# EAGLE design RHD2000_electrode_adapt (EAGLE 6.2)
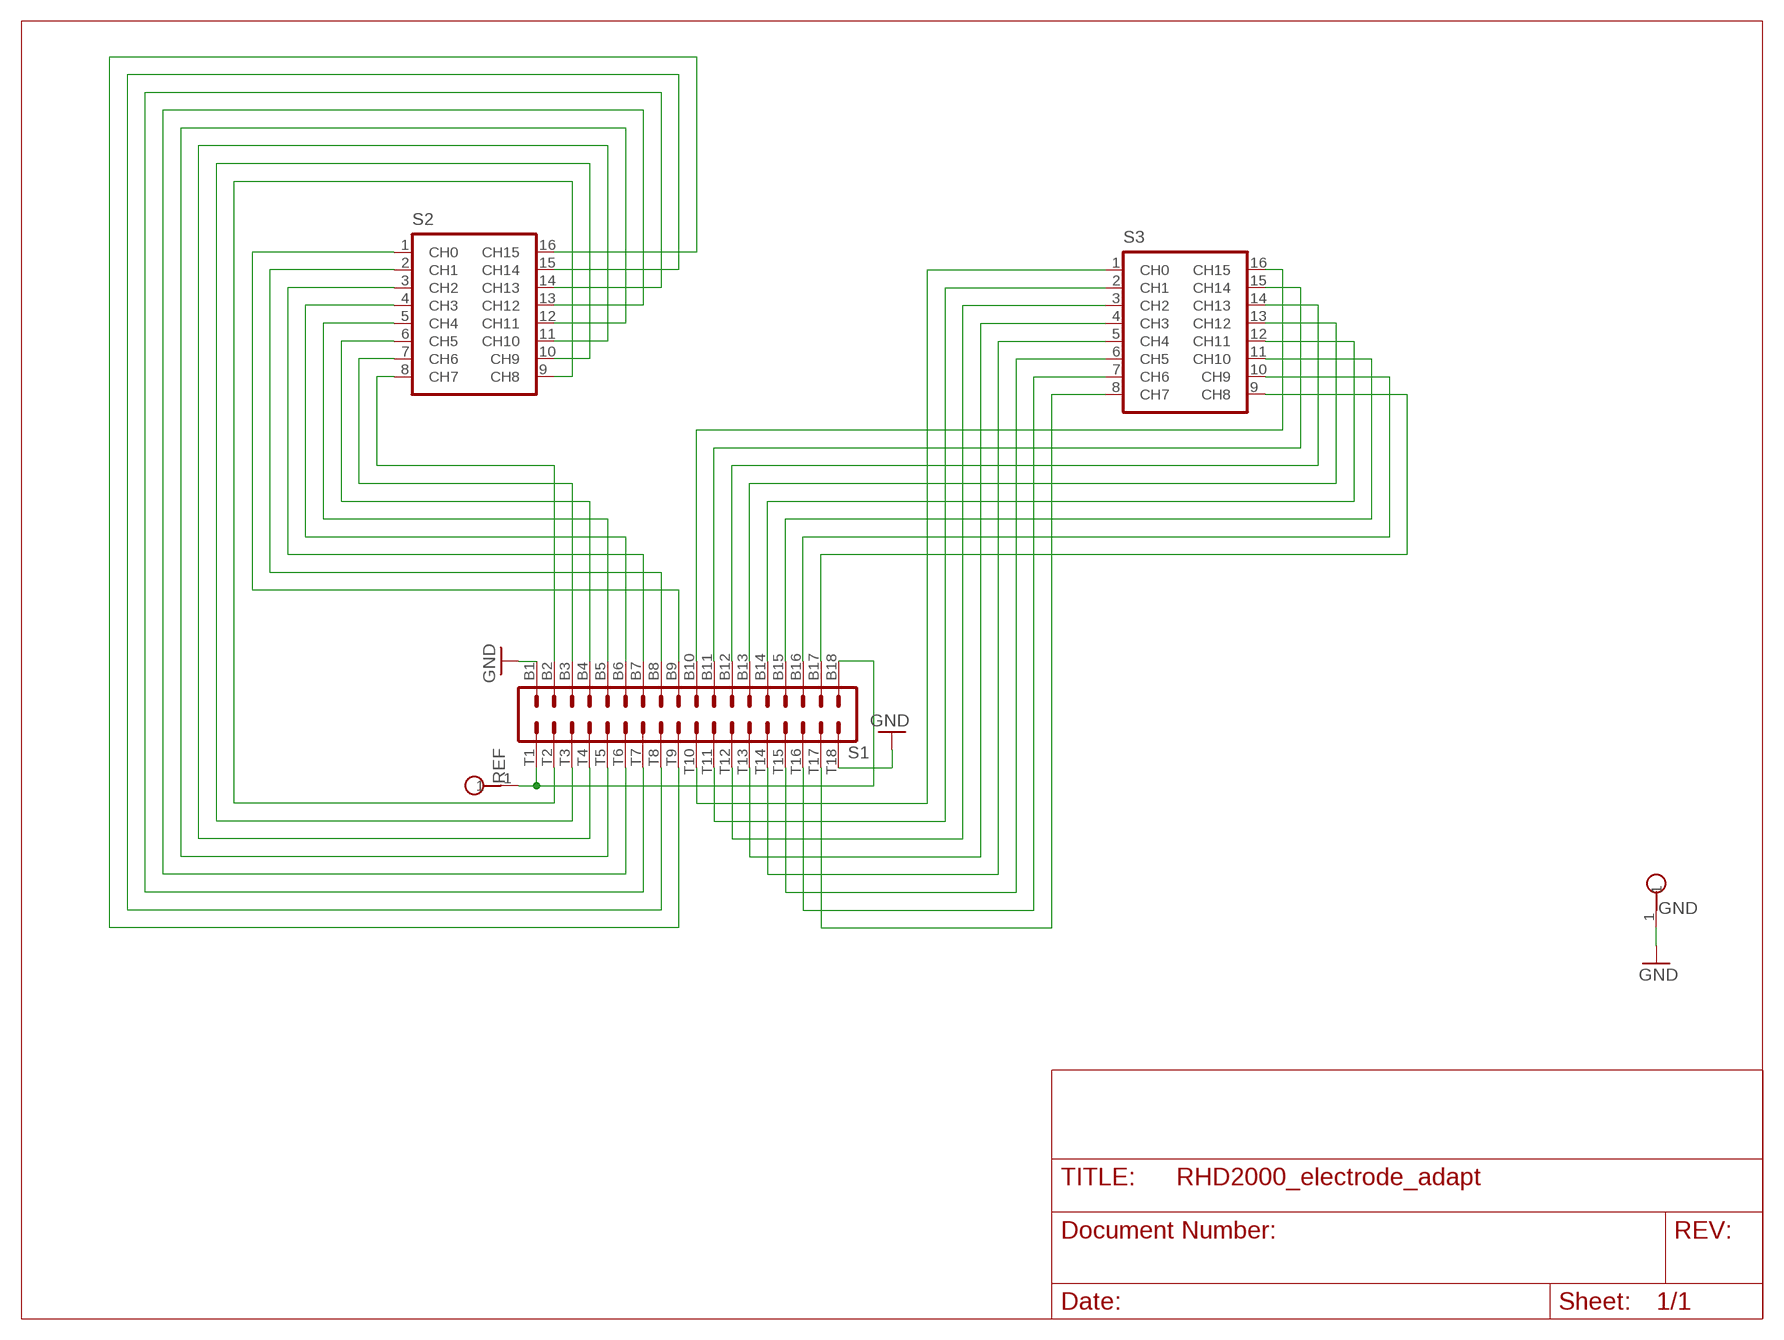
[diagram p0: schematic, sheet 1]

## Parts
GND  TESTPOINT_SMALL  [TESTPOINT_SMALL]
REF  TESTPOINT_SMALL  [TESTPOINT_SMALL]
S1  OMNETICS_A79024  [OMNETICS_A79024]
S2  DIP16_SOCKET  [DIL16_SOCKET]
S3  DIP16_SOCKET  [DIL16_SOCKET]

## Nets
GND: GND.1 S1.B1 S1.T18
N$1: REF.1 S1.B18 S1.T1
N$2: S1.B2 S2.8(CH7)
N$3: S1.B3 S2.7(CH6)
N$4: S1.B4 S2.6(CH5)
N$5: S1.B5 S2.5(CH4)
N$6: S1.B6 S2.4(CH3)
N$7: S1.B7 S2.3(CH2)
N$8: S1.B8 S2.2(CH1)
N$9: S1.B9 S2.1(CH0)
N$10: S1.T2 S2.9(CH8)
N$11: S1.T3 S2.10(CH9)
N$12: S1.T4 S2.11(CH10)
N$13: S1.T5 S2.12(CH11)
N$14: S1.T6 S2.13(CH12)
N$15: S1.T7 S2.14(CH13)
N$16: S1.T8 S2.15(CH14)
N$17: S1.T9 S2.16(CH15)
N$18: S1.T10 S3.1(CH0)
N$19: S1.T11 S3.2(CH1)
N$20: S1.T12 S3.3(CH2)
N$21: S1.T13 S3.4(CH3)
N$22: S1.T14 S3.5(CH4)
N$23: S1.T15 S3.6(CH5)
N$24: S1.T16 S3.7(CH6)
N$25: S1.T17 S3.8(CH7)
N$26: S1.B10 S3.16(CH15)
N$27: S1.B11 S3.15(CH14)
N$28: S1.B12 S3.14(CH13)
N$29: S1.B13 S3.13(CH12)
N$30: S1.B14 S3.12(CH11)
N$31: S1.B15 S3.11(CH10)
N$32: S1.B16 S3.10(CH9)
N$33: S1.B17 S3.9(CH8)

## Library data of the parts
GND REF = RHD2000_eval_board:TESTPOINT: PCB Test Point
S1 = RHD2000_eval_board:OMNETICS_A79024: Omnetics A79024 36-pin connector
S2 S3 = RHD2000_eval_board:DIP16_SOCKET: DIP-16 socket footprint

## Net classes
1 thick: width 1.016 mm
2 power: width 0.61 mm

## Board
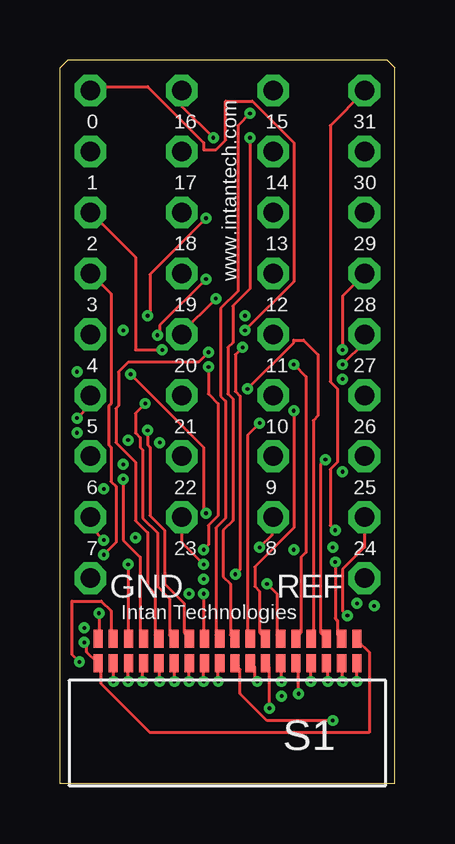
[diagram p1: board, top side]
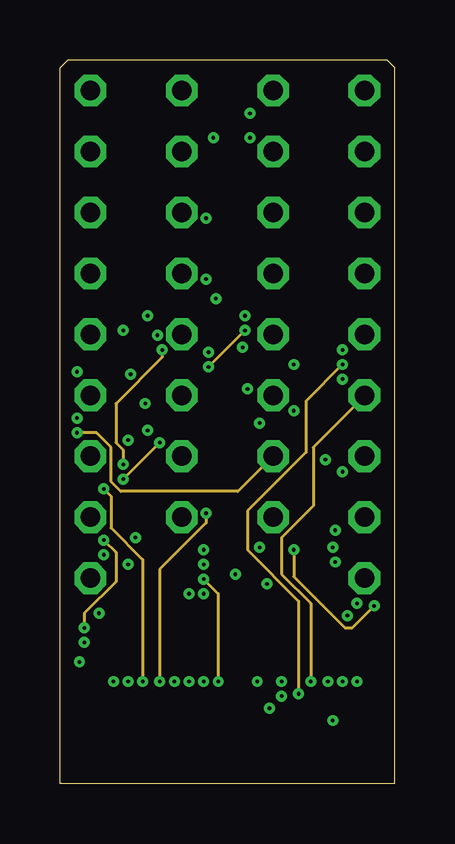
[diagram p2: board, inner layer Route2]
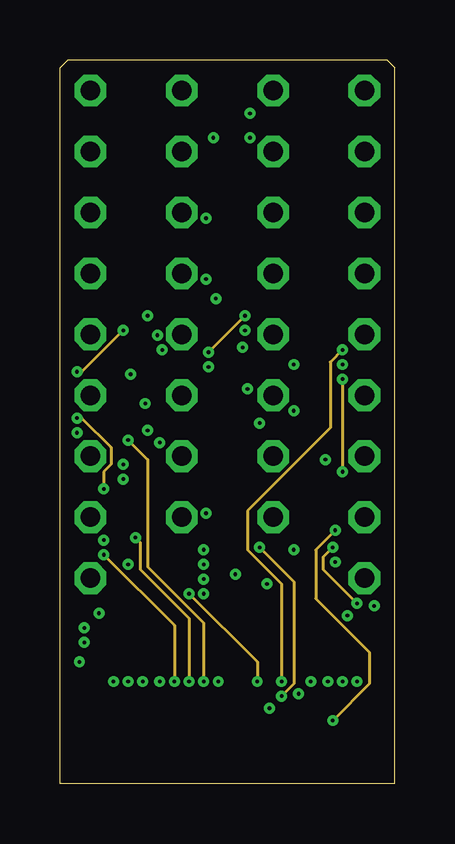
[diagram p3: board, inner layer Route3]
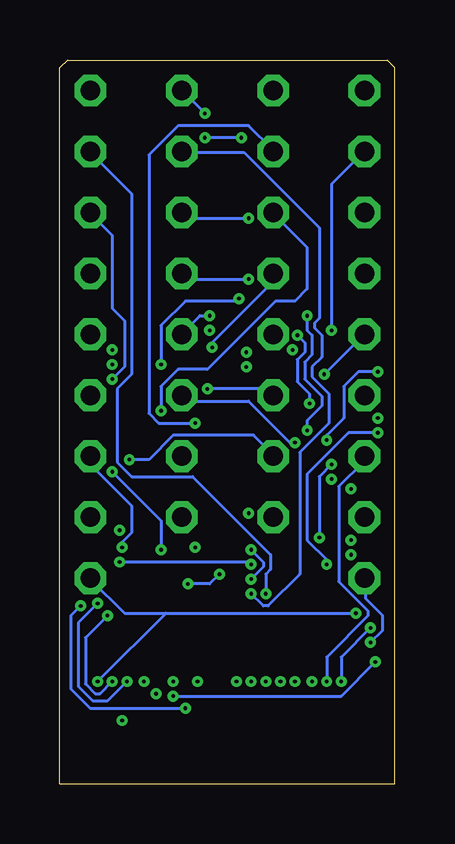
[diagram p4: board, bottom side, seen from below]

Size 13.97 x 30.16 mm. Coordinates in mm from the lower left corner, seen from the top.
Outline: 0,0 0,29.84 0.32,30.16 13.65,30.16 13.97,29.84 13.97,0 0,0
Copper layers (1*2+3*16): Top 0.035mm / dielectric 1.5mm / Route2 0.035mm / dielectric 0.15mm / Route3 0.035mm / dielectric 0.2mm / Bottom 0.035mm
Design rules: minimum track width 5mil, minimum drill 6mil, track to track 5mil, track to pad 5mil, pad to pad 5mil, via to via 5mil, smd to smd 5mil, copper to edge 15mil, drill to drill 15mil, minimum pad ring 10mil, minimum via ring 6mil, stop-mask expansion 4mil, vias tented up to drill 0mil, thermal gap 10mil
vRestrict: area 2.2,7.6 to 5.1,8.9; area 8.9,7.6 to 11.7,8.9; area 12.1,9.5 to 13.3,10.2; area 12.1,12.1 to 13.3,12.7; area 12.1,14.6 to 13.3,15.2; area 12.1,17.1 to 13.3,17.8; area 12.1,19.7 to 13.3,20.3; area 12.1,22.2 to 13.3,22.9; area 12.1,24.8 to 13.3,25.4; area 12.1,27.3 to 13.3,27.9; area 8.6,27.3 to 9.5,27.9; area 8.6,24.8 to 9.5,25.4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

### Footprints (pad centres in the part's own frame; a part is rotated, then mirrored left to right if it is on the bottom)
TESTPOINT_SMALL = drill 0.813 octagon: 1 0,0
OMNETICS_A79024 = smd 0.381 x 0.762: B1 -5.397,0.711; B2 -4.763,0.711; B3 -4.128,0.711; B4 -3.493,0.711; B5 -2.857,0.711; B6 -2.223,0.711; B7 -1.587,0.711; B8 -0.953,0.711; B9 -0.318,0.711; B10 0.318,0.711; B11 0.953,0.711; B12 1.587,0.711; B13 2.223,0.711; B14 2.857,0.711; B15 3.493,0.711; B16 4.128,0.711; B17 4.763,0.711; B18 5.397,0.711; T1 -5.397,1.727; T2 -4.763,1.727; T3 -4.128,1.727; T4 -3.493,1.727; T5 -2.857,1.727; T6 -2.223,1.727; T7 -1.587,1.727; T8 -0.953,1.727; T9 -0.318,1.727; T10 0.318,1.727; T11 0.953,1.727; T12 1.587,1.727; T13 2.223,1.727; T14 2.857,1.727; T15 3.493,1.727; T16 4.128,1.727; T17 4.763,1.727; T18 5.397,1.727
DIL16_SOCKET = drill 0.813 octagon: 1 -7.62,-3.81; 2 -5.08,-3.81; 3 -2.54,-3.81; 4 0,-3.81; 5 2.54,-3.81; 6 5.08,-3.81; 7 7.62,-3.81; 8 10.16,-3.81; 9 10.16,3.81; 10 7.62,3.81; 11 5.08,3.81; 12 2.54,3.81; 13 0,3.81; 14 -2.54,3.81; 15 -5.08,3.81; 16 -7.62,3.81

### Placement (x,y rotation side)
GND  1.27,8.57 180 top
REF  12.7,8.57 180 top
S1  6.99,4.32 0 top
S2  5.08,21.27 270 top
S3  8.89,21.27 270 top

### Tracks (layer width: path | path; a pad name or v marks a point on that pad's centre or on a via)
GND  (via drill 0.15)
  Top 0.127: S1.T18 12.39,5.99 12.9,5.49 12.9,2.13 3.76,2.13 1.73,4.17 1.73,4.88 1.63,4.98 S1.B1 1.52,5.08 1.12,5.49 1.12,5.79 v1.02,5.89
  Bottom 0.127: v1.02,5.89 0.51,6.4 0.51,7.01 1.22,7.72 1.22,8.53 GND.1
N$1  (via drill 0.15)
  Top 0.127: v1.63,7.11 1.63,6.1 S1.T1 | v12.39,4.27 12.39,4.98 S1.B18
  Bottom 0.127: 9.55,7.11 11.28,7.11 12.7,8.53 REF.1 | 9.55,7.11 v1.63,7.11 | 9.55,7.11 v12.39,4.27
N$2  (via drill 0.15)
  Top 0.127: v2.23,4.27 2.23,4.98 S1.B2 | v1.83,10.16 1.32,10.67 1.32,11.07 S2.8
  Route2 0.127: v1.02,6.5 1.02,7.11 2.34,8.43 2.34,9.65 v1.83,10.16
  Bottom 0.127: v2.23,4.27 2.23,5.28 v1.02,6.5
N$3  (via drill 0.15)
  Top 0.127: v2.85,4.27 2.85,4.98 S1.B3
  Bottom 0.127: v2.85,4.27 2.85,5.28 1.12,7.01 1.12,7.21 2.34,8.43 2.34,12.39 1.32,13.41 1.32,13.61 S2.7
N$4  (via drill 0.15)
  Top 0.127: v3.45,4.27 3.45,4.98 S1.B4 | v0.71,15.24 1.22,15.75 1.22,16.15 S2.6
  Route2 0.127: v3.45,4.27 3.45,9.35 2.13,10.67 2.13,11.99 v1.83,12.29
  Route3 0.127: v1.83,12.29 1.83,13.01 2.13,13.31 2.13,14.02 0.91,15.24 v0.71,15.24
N$5  (via drill 0.15)
  Top 0.127: v4.17,4.27 4.17,4.98 S1.B5 | v6.1,11.28 5.99,11.38 5.99,14.02 v2.95,17.07
  Route2 0.127: v4.17,4.27 4.17,8.94 6.1,10.87 v6.1,11.28
  Bottom 0.127: v2.95,17.07 1.32,18.69 S2.5
N$6  (via drill 0.15)
  Top 0.127: v4.78,4.27 4.78,4.98 S1.B6 | v1.83,9.55 2.34,10.06 2.34,12.39 2.13,12.6 2.13,14.02 2.03,14.12 2.03,15.75 2.13,15.85 2.13,20.42 1.32,21.23 S2.4
  Route3 0.127: v4.78,4.27 4.78,6.6 v1.83,9.55
N$7  (via drill 0.15)
  Top 0.127: v5.38,4.27 5.38,4.98 S1.B7 | v4.27,18.09 3.15,18.09 3.15,21.95 1.32,23.77 S2.3
  Route2 0.127: v2.64,13.31 2.64,13.92 2.34,14.22 2.34,15.85 4.27,17.78 v4.27,18.09
  Route3 0.127: v5.38,4.27 5.38,6.91 3.35,8.94 3.35,10.06 v3.15,10.26
  Bottom 0.127: v3.15,10.26 3.15,12.8 v2.64,13.31
N$8  (via drill 0.15)
  Top 0.127: v5.99,4.27 5.99,4.98 S1.B8
  Route3 0.127: v5.99,4.27 5.99,6.71 3.66,9.04 3.66,13.51 v2.85,14.33 | v0.71,17.17 0.91,17.17 v2.64,18.9
  Bottom 0.127: v2.85,14.33 2.85,14.53 2.13,15.24 2.13,16.56 1.52,17.17 v0.71,17.17 | v2.64,18.9 2.64,24.99 1.32,26.31 S2.2
N$9  (via drill 0.15)
  Top 0.127: v6.6,4.27 6.6,4.98 S1.B9 | v5.99,9.75 6.2,9.96 6.2,10.77 6.6,11.18 6.6,15.85 6.2,16.26 v6.2,17.37 | v7.72,18.9 9.75,20.93 9.75,26.72 8.03,28.45 6.91,28.45 6.91,26.82 6.5,26.42 5.99,26.42 5.99,26.72 3.66,29.06 1.32,29.06 1.32,28.96 S2.1
  Route2 0.127: v6.6,4.27 6.6,7.92 v5.99,8.53 | v7.72,18.9 v6.2,17.37
  Bottom 0.127: v5.99,8.53 5.49,9.04 5.49,9.25 v5.99,9.75
N$10  (via drill 0.15)
  Top 0.127: v0.81,5.08 0.51,5.38 0.51,7.62 1.73,7.62 2.13,7.21 2.13,6.1 S1.T2 | v8.33,9.86 8.84,10.36 8.84,11.07 S2.9
  Route3 0.127: v9.25,3.66 9.75,4.17 9.75,8.43 v8.33,9.86
  Bottom 0.127: v0.81,5.08 2.23,3.66 v9.25,3.66
N$11  (via drill 0.15)
  Top 0.127: v2.85,9.14 2.85,6.1 S1.T3
  Route2 0.127: v0.71,14.63 1.52,14.63 2.13,14.02 2.13,12.6 2.54,12.19 7.42,12.19 8.84,13.61 S2.10
  Bottom 0.127: v2.85,9.14 2.85,9.35 3.66,10.16 3.66,12.9 1.93,14.63 v0.71,14.63
N$12  (via drill 0.15)
  Top 0.127: v2.64,12.7 2.64,10.16 3.35,9.45 3.35,6.2 3.45,6.1 S1.T4
  Route2 0.127: v4.17,14.22 v2.64,12.7
  Bottom 0.127: v4.17,14.22 4.37,14.22 6.1,15.95 8.64,15.95 8.84,16.15 S2.11
N$13  (via drill 0.15)
  Top 0.127: v6.2,17.98 5.79,17.58 2.85,17.58 2.44,17.17 2.44,15.75 2.34,15.65 2.34,14.22 3.15,13.41 3.15,10.97 3.66,10.46 3.66,8.23 3.96,7.92 3.96,6.2 4.06,6.1 S1.T5
  Route3 0.127: v7.72,19.51 v6.2,17.98
  Bottom 0.127: v7.72,19.51 8.13,19.51 8.84,18.8 S2.12
N$14  (via drill 0.15)
  Top 0.127: v3.56,15.85 3.15,15.44 3.15,14.63 3.35,14.43 3.35,14.02 3.45,13.92 3.45,11.07 4.06,10.46 4.06,8.23 4.57,7.72 4.57,6.2 4.67,6.1 S1.T6 | v4.06,18.69 4.17,18.8 4.17,19.1 v6.1,21.03
  Bottom 0.127: v3.56,15.85 3.56,16.26 4.06,16.76 4.06,17.68 3.76,17.98 3.76,18.39 v4.06,18.69 | v6.1,21.03 8.64,21.03 8.84,21.23 S2.13
N$15  (via drill 0.15)
  Top 0.127: v3.66,14.73 3.66,14.12 3.76,14.02 3.76,11.18 4.37,10.57 4.37,8.33 5.18,7.52 5.18,6.3 5.38,6.1 S1.T7 | v3.66,19.51 3.76,19.61 3.76,21.23 v6.1,23.57
  Bottom 0.127: v3.66,14.73 3.66,15.14 3.05,15.75 3.05,16.15 3.76,16.87 3.76,17.58 3.45,17.88 3.45,18.69 3.66,18.9 v3.66,19.51 | v6.1,23.57 8.64,23.57 8.84,23.77 S2.14
N$16  (via drill 0.15)
  Top 0.127: v5.99,7.92 5.99,6.1 S1.T8
  Bottom 0.127: v5.99,7.92 5.49,7.42 5.28,7.42 3.96,8.74 3.96,13.82 2.74,15.04 2.74,16.26 3.45,16.97 3.45,17.37 3.05,17.78 3.05,18.69 3.35,19 3.35,19.2 3.15,19.41 3.15,23.16 6.3,26.31 8.84,26.31 S2.15
N$17  (via drill 0.15)
  Top 0.127: v7.92,27.94 7.42,27.43 7.42,20.52 6.71,19.81 6.71,16.15 6.91,15.95 6.91,11.07 6.5,10.67 6.5,6.2 6.6,6.1 S1.T9
  Bottom 0.127: v7.92,27.94 8.84,28.85 S2.16
N$18  (via drill 0.15)
  Top 0.127: v7.92,26.92 7.92,20.62 7.21,19.91 7.21,18.39 7.01,18.19 7.01,16.26 7.21,16.05 7.21,10.97 6.81,10.57 6.81,8.64 7.11,8.33 7.11,6.2 7.21,6.1 S1.T10 | v6.4,26.92 5.08,28.25 S3.1
  Bottom 0.127: v6.4,26.92 v7.92,26.92
N$19  (via drill 0.15)
  Top 0.127: v8.33,15.04 7.82,14.53 7.82,6.2 7.92,6.1 S1.T11
  Bottom 0.127: v8.33,15.04 9.86,15.04 10.26,15.44 10.26,26.21 9.04,27.43 6.1,27.43 5.08,26.42 S3.2
N$20  (via drill 0.15)
  Top 0.127: v9.75,15.54 9.75,10.67 8.13,9.04 8.13,8.23 8.33,8.03 8.33,6.3 8.53,6.1 S1.T12
  Bottom 0.127: v9.75,15.54 9.75,16.56 9.04,17.27 7.82,17.27 4.98,20.12 4.17,20.12 3.66,20.62 3.66,22.35 5.08,23.77 S3.3
N$21  (via drill 0.15)
  Top 0.127: v8.64,8.33 9.04,7.92 9.04,6.2 9.14,6.1 S1.T13 | v7.32,8.74 7.52,8.94 7.52,16.15 7.32,16.36 7.32,17.88 v7.62,18.19
  Bottom 0.127: v8.64,8.33 7.72,8.33 v7.32,8.74 | v7.62,18.19 7.62,18.39 5.08,20.93 S3.4
N$22  (via drill 0.15)
  Top 0.127: v9.75,17.48 10.26,16.97 10.26,9.65 10.06,9.45 10.06,6.3 9.86,6.1 S1.T14 | v6.5,20.22 5.08,18.8 S3.5
  Bottom 0.127: v9.75,17.48 9.75,19.1 8.74,20.12 6.6,20.12 v6.5,20.22
N$23  (via drill 0.15)
  Top 0.127: v7.82,16.46 9.75,18.39 9.75,18.49 10.16,18.49 10.77,17.88 10.77,15.34 10.57,15.14 10.57,6.1 S1.T15
  Bottom 0.127: v7.82,16.46 5.28,16.46 5.08,16.26 S3.6
N$24  (via drill 0.15)
  Top 0.127: v11.07,13.51 10.87,13.31 10.87,6.3 11.07,6.1 S1.T16
  Bottom 0.127: v11.07,13.51 10.26,13.51 9.25,14.53 5.89,14.53 5.08,13.72 S3.7
N$25  (via drill 0.15)
  Top 0.127: v11.48,9.25 11.48,6.91 11.58,6.81 11.58,6.2 11.68,6.1 S1.T17 | v5.99,9.14 5.08,10.06 S3.8
  Bottom 0.127: v11.48,9.25 6.1,9.25 v5.99,9.14
N$26  (via drill 0.15)
  Top 0.127: v11.38,2.64 8.64,2.64 7.52,3.76 7.52,4.78 7.32,4.98 S1.B10 | v11.48,10.57 11.28,10.77 11.28,13.11 11.58,13.41 11.58,16.46 11.28,16.76 11.28,27.43 12.7,28.85 S3.16
  Route3 0.127: v11.38,2.64 12.9,4.17 12.9,5.49 10.67,7.72 10.67,9.75 v11.48,10.57
N$27  (via drill 0.15)
  Top 0.127: v8.23,4.27 8.13,4.37 8.13,4.88 8.03,4.98 S1.B11
  Route3 0.127: v8.23,4.27 8.23,5.08 v5.38,7.92
  Bottom 0.127: v5.38,7.92 5.38,8.74 5.18,8.94 5.18,9.55 8.43,12.8 10.97,12.8 11.58,13.41 11.58,16.46 10.97,17.07 10.97,24.59 12.7,26.31 S3.15
N$28  (via drill 0.15)
  Top 0.127: v8.74,3.15 8.74,4.88 8.64,4.98 S1.B12
  Route2 0.127: v13.11,7.42 12.19,6.5 11.89,6.5 9.75,8.64 v9.75,9.75
  Route3 0.127: v11.79,16.87 v11.79,13.01
  Bottom 0.127: v8.74,3.15 12.7,3.15 13.51,3.96 13.51,7.01 v13.11,7.42 | v9.75,9.75 9.75,10.97 v11.79,13.01 | v11.79,16.87 11.28,17.37 11.28,19.3 11.79,19.81 11.79,22.86 12.7,23.77 S3.14
N$29  (via drill 0.15)
  Top 0.127: v9.25,4.27 9.25,4.98 S1.B13 | v11.79,18.09 11.79,20.32 12.7,21.23 S3.13
  Route3 0.127: v9.25,4.27 9.25,8.33 7.82,9.75 7.82,11.38 11.28,14.83 11.28,17.58 v11.79,18.09
N$30  (via drill 0.15)
  Top 0.127: v9.96,3.76 9.96,4.88 9.86,4.98 S1.B14 | v11.79,17.48 12.7,18.39 S3.12
  Route2 0.127: v9.96,3.76 9.96,7.62 7.82,9.75 7.82,11.38 10.26,13.82 10.26,15.95 v11.79,17.48
N$31  (via drill 0.15)
  Top 0.127: v10.46,4.27 10.46,4.98 S1.B15
  Route2 0.127: v10.46,4.27 10.46,7.52 9.25,8.74 9.25,10.26 10.57,11.58 10.57,14.02 12.7,16.15 S3.11
N$32  (via drill 0.15)
  Top 0.127: v11.18,4.27 11.18,4.98 S1.B16
  Route3 0.127: v12.39,7.52 10.97,8.94 10.97,9.45 v11.38,9.86
  Bottom 0.127: v11.18,4.27 11.99,3.45 12.6,3.45 13.21,4.06 13.21,6.71 v12.39,7.52 | v11.38,9.86 11.38,10.06 10.97,10.46 10.97,11.58 12.7,13.31 S3.10
N$33  (via drill 0.15)
  Top 0.127: v11.79,4.27 11.79,4.98 S1.B17 | v11.99,7.01 11.79,7.21 11.79,8.94 12.7,9.86 S3.9
  Bottom 0.127: v11.79,4.27 12.29,3.76 12.5,3.76 12.9,4.17 12.9,6.1 v11.99,7.01

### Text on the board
tPlace: 0 | 16 | 15 | 31 | 1 | 17 | 14 | 30 | 2 | 18 | 13 | 29 | www.intantech.com | 3 | 19 | 12 | 28 | 4 | 20 | 11 | 27 | 5 | 21 | 10 | 26 | 6 | 22 | 9 | 25 | 7 | 23 | 8 | 24 | Intan Technologies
